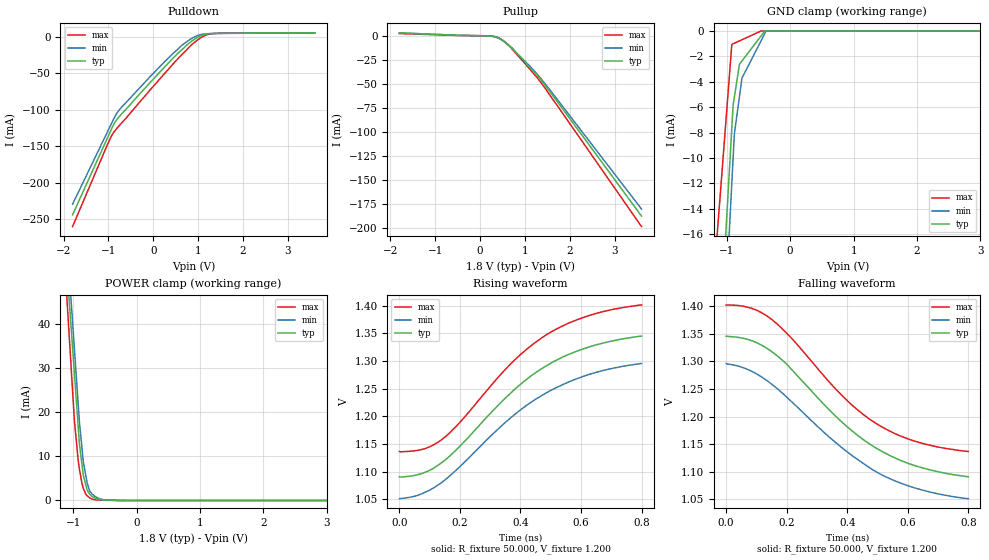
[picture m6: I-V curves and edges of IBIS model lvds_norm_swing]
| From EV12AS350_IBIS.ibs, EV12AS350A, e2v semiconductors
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[Model]   lvds_norm_swing
Model_type Output
Vref=1.200E+00
Rref=5.000E+01
Cref=5.000E-12
Vmeas=1.200E+00
C_comp   8.430E-13   7.910E-13   8.950E-13
[Voltage Range]   1.800E+00   1.700E+00   1.900E+00
[POWER Clamp Reference]   1.800E+00   1.700E+00   1.900E+00
[GND Clamp Reference]   0.000E+00   0.000E+00   0.000E+00
[Pullup Reference]   1.800E+00   1.700E+00   1.900E+00
[Pulldown Reference]   0.000E+00   0.000E+00   0.000E+00
[Temperature Range]   25   110   -40
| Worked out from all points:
|   slope of the pulldown table from 0 to 0.27 V, typ, clamps not added: 15.2 ohm
|   slope of the pullup table from 0 to 0.27 V, typ, clamps not added: 438 ohm
|   POWER clamp passes 1 mA (typ) near -0.71 V on its own axis
|   rising waveform, R_fixture 50.000, V_fixture 1.200: 20-80 % time 302ps typ, 317ps min, 288ps max; typ from 1.09 V to 1.34 V
|   falling waveform, R_fixture 50.000, V_fixture 1.200: 20-80 % time 298ps typ, 319ps min, 285ps max; typ from 1.34 V to 1.09 V
[GND Clamp]
-1.9V     -93.59mA   -106.3mA   -64.52mA
-1.7V     -76.04mA   -87.07mA   -51.56mA
-920mV    -7.599mA   -11.95mA   -1.051mA
-900mV    -5.844mA   -10.03mA   -1.005mA
-880mV    -5.2mA     -8.101mA   -959.4uA
-800mV    -2.622mA   -5.171mA   -776.6uA
-760mV    -2.36mA    -3.706mA   -685.3uA
-460mV    -393.3uA   -780.3uA   0A
-400mV    0A         -195.1uA   0A
-380mV    0A         0A         0A
3.8V      0A         0A         0A
[POWER Clamp]
-2V       234.4mA    247.2mA    256.5mA
-1.6V     153.8mA    163.8mA    163mA
-1.08V    48.9mA     55.2mA     41.46mA
-1.02V    36.8mA     42.68mA    27.44mA
-980mV    28.74mA    34.33mA    18.09mA
-920mV    16.64mA    21.8mA     9.019mA
-900mV    12.61mA    17.63mA    6.948mA
-840mV    5.787mA    8.818mA    2.787mA
-740mV    1.428mA    2.15mA     608uA
-560mV    167uA      293uA      92.95uA
-280mV    0A         6.917uA    0A
3.7V      0A         0A         0A
[Pullup]
-1.8V     3.525mA    3.383mA    2.731mA
240mV     83.42uA    61.82uA    197.1uA
400mV     -1.617mA   -1.82mA    -1.38mA
540mV     -5.571mA   -5.731mA   -5.526mA
740mV     -13.9mA    -13.57mA   -14.72mA
1.12V     -32.83mA   -31.61mA   -34.89mA
1.38V     -46.96mA   -45.53mA   -49.72mA
3.6V      -187.3mA   -179.9mA   -198.2mA
[Pulldown]
-1.8V     -244.5mA   -229.8mA   -260.5mA
-1.02V    -138.5mA   -130.2mA   -147.6mA
-900mV    -122.4mA   -114.9mA   -132.8mA
-820mV    -114.2mA   -105.6mA   -126.3mA
-720mV    -106.7mA   -97.57mA   -119.2mA
160mV     -47.5mA    -39.97mA   -56.82mA
640mV     -17.65mA   -11.69mA   -24.29mA
920mV     -3.337mA   -93.98uA   -7.572mA
1.04V     924.3uA    2.803mA    -2.058mA
1.16V     3.418mA    3.998mA    1.921mA
1.36V     4.599mA    4.58mA     4.497mA
3.6V      5.426mA    5.464mA    5.444mA
[Rising Waveform]
R_fixture = 50.000
V_fixture = 1.200
V_fixture_min = 1.200
V_fixture_max = 1.200
|  time   V(typ)   V(min)   V(max)
0s        1.091V     1.051V     1.137V
85ps      1.099V     1.063V     1.142V
145ps     1.119V     1.083V     1.16V
205ps     1.149V     1.112V     1.192V
370ps     1.243V     1.199V     1.296V
435ps     1.273V     1.226V     1.328V
495ps     1.294V     1.246V     1.351V
555ps     1.311V     1.261V     1.368V
630ps     1.326V     1.276V     1.383V
800ps     1.345V     1.296V     1.402V
[Falling Waveform]
R_fixture = 50.000
V_fixture = 1.200
V_fixture_min = 1.200
V_fixture_max = 1.200
|  time   V(typ)   V(min)   V(max)
0s        1.345V     1.296V     1.402V
80ps      1.338V     1.283V     1.396V
150ps     1.318V     1.259V     1.376V
220ps     1.283V     1.225V     1.339V
325ps     1.221V     1.17V      1.272V
395ps     1.184V     1.138V     1.231V
450ps     1.159V     1.116V     1.205V
505ps     1.14V      1.097V     1.184V
625ps     1.111V     1.071V     1.155V
800ps     1.091V     1.051V     1.137V
[Ramp]
dV/dt_r   1.5792E-01/3.0220E-10   1.4664E-01/3.1730E-10   1.5894E-01/2.8810E-10
dV/dt_f   1.5792E-01/2.9806E-10   1.4664E-01/3.1860E-10   1.5894E-01/2.8536E-10
R_load = 50
